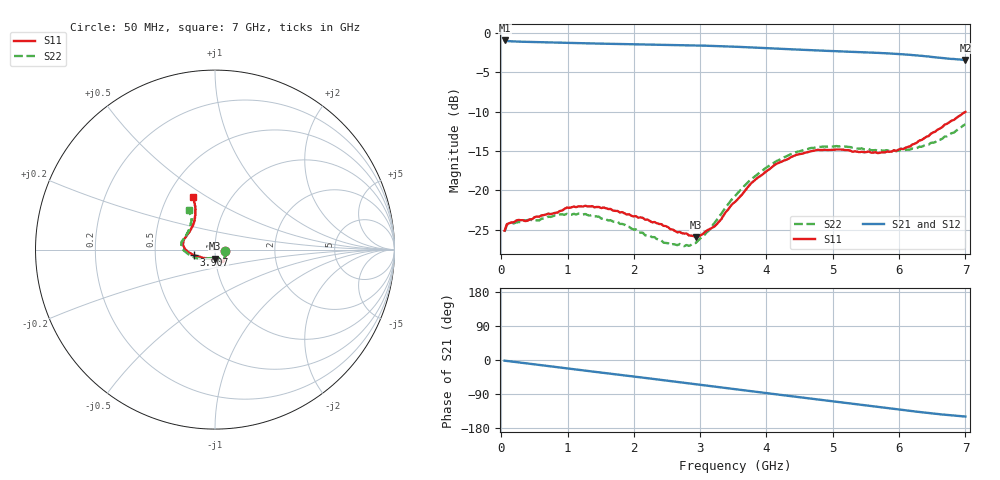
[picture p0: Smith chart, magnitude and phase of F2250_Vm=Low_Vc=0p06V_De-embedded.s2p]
! Integrated Device Technology
! Corporate Headquarters
! 6024 Silver Creek Valley Road
! San Jose, CA 95138  USA
! Phone:  1-408-284-8200
! Toll Free:  1-800-223-1366
! Webpage:  http://www.idt.com/
! Timing and RF Division
! 515 Groton Road, Suite 102
! Westford, MA 01886-6024
! Device:  F2250
! Description: Voltage Variable RF Attenuator
! Frequency:  50.0 -  6000.00 MHz
! Package:  3x3 mm Thin QFN Plastic Package: 16 pin
! Ports:  2 RF, 3 DC
!  Pin  1  = GND
!  Pin  2  = NC
!  Pin  3  = RF1  = Port 1
!  Pin  4  = NC
!  Pin  5  = GND
!  Pin  6  = GND
!  Pin  7  = GND
!  Pin  8  = GND
!  Pin  9  = NC
!  Pin 10  = RF2  = Port 2
!  Pin 11  = NC
!  Pin 12  = GND
!  Pin 13  = GND
!  Pin 14  = VCNTRL
!  Pin 15  = VDD
!  Pin 16  = VMODE
! Vcntrl:  0.060 Volts
! Vmode:  +0.000 Volts
! Vdd:  +3.30  Volts
! Current:  1.106 mA
! Data:  The device was measured on a the F2250 evaluation board which has
!  individual transmission lines to the RF pins.  Data was collected
!  using a calibrated network analyzer.  The evaluation board was
!  de-embedded using a TRL calibration technique.
!  The reference plane is the edge of the package pin.
! Misc:  SN 10
!  Action Tracker AT0258
! Date Measured:  2014-11-26
! Date:  2015-10-15  MJV
! Note:
!  Integrated Device Technology supplies this data as a sample of measured
!  data at the package pin for this product.  Your particular data for this
!  product may vary.
!  Data was taken at 25 degrees C.
!  Integrated Device Technology reserves the right to change this data at anytime.
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# GHz S dB R 50
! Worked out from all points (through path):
!   201 points, 50 MHz to 7 GHz, reference 50 ohm
!   highest |S21| = -0.93 dB at 50 MHz (marker M1); lowest = -3.4 dB at 7 GHz (marker M2)
!   group delay of S21, straight-line fit = 59.9 ps
!   lowest |S11| = -26.0 dB at 2.934 GHz (marker M3), VSWR 1.11, Z = 49.5 - j4.99 ohm
!   |S11| at or under -10 dB: start of sweep to end of sweep
!   |S22| runs from -27.1 to -11.6 dB; largest |S21 - S12| = 0.00029
!   S11 on the Smith chart (normalised r, x): 50 MHz: 1.12, -0.02; 3.907 GHz: 0.79, -0.05; 7 GHz: 0.67, +0.43
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0.05  -25.12 -9.7  -0.93 -1.8  -0.93 -1.8  -25.23 -10.1
0.08475  -24.29 -9.7  -0.99 -2.5  -0.99 -2.5  -24.35 -9.4
0.15425  -24.07 -11.9  -1.04 -4.0  -1.04 -3.9  -24.10 -11.0
0.57125  -23.35 -30.1  -1.14 -13.1  -1.14 -13.1  -23.82 -30.4
0.884  -22.62 -45.9  -1.20 -19.9  -1.20 -19.9  -23.05 -46.8
1.2315  -22.06 -56.0  -1.28 -27.4  -1.28 -27.3  -23.06 -59.7
1.75275  -22.62 -62.8  -1.37 -38.4  -1.37 -38.4  -23.96 -66.7
2.37825  -24.27 -63.6  -1.46 -51.8  -1.46 -51.8  -26.30 -67.8
2.552  -24.95 -67.8  -1.49 -55.6  -1.49 -55.6  -26.95 -73.3
2.83  -25.72 -83.3  -1.54 -61.7  -1.54 -61.7  -27.06 -92.7
2.93425  -25.97 -92.5  -1.56 -64.0  -1.56 -64.0  -26.68 -101.5
3.21225  -24.62 -122.1  -1.63 -70.1  -1.63 -70.1  -24.17 -127.6
3.525  -21.47 -148.3  -1.72 -77.0  -1.72 -77.0  -20.72 -146.4
3.76825  -19.09 -161.3  -1.81 -82.4  -1.81 -82.4  -18.56 -156.7
3.90725  -18.18 -165.6  -1.87 -85.4  -1.87 -85.4  -17.67 -162.8
4.1505  -16.61 -173.7  -1.97 -90.7  -1.96 -90.7  -16.27 -171.4
4.7065  -14.96 172.3  -2.18 -102.7  -2.18 -102.7  -14.60 175.7
5.15825  -14.82 161.5  -2.33 -112.5  -2.33 -112.4  -14.37 166.6
5.85325  -15.10 138.4  -2.58 -127.4  -2.58 -127.4  -15.00 151.6
6.166  -14.40 127.6  -2.75 -134.2  -2.75 -134.2  -14.81 142.8
6.444  -13.10 119.3  -2.96 -140.0  -2.96 -140.0  -14.19 133.4
7  -10.01 113.1  -3.41 -149.2  -3.41 -149.2  -11.60 123.9
